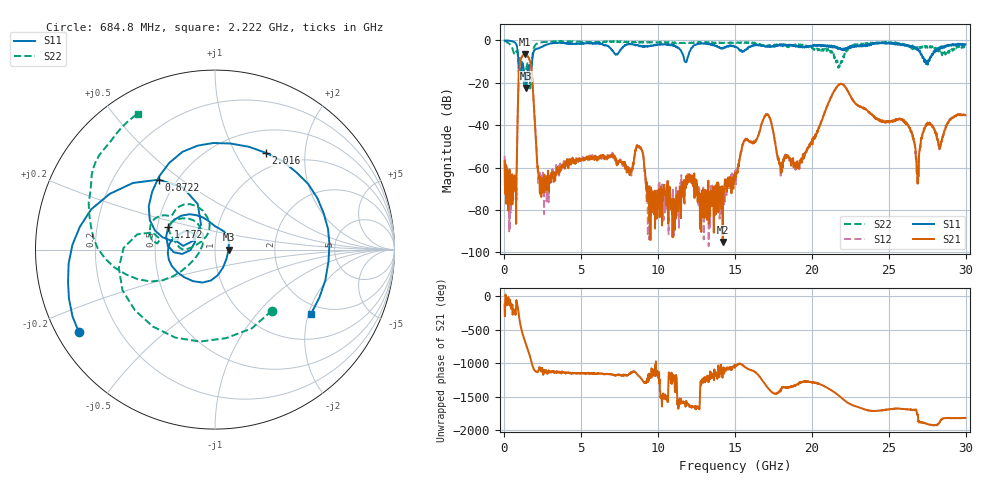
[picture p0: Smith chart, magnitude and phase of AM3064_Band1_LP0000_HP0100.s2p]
# Hz S DB R 50.0
!freq dBS11 angS11 dBS21 angS21 dBS12 angS12 dBS22 angS22
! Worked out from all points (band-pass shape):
!   1600 points, 10 MHz to 29.98 GHz, reference 50 ohm
!   highest |S21| = -6.49 dB at 1.322 GHz (marker M1); lowest = -95.1 dB at 14.2 GHz (marker M2)
!   |S21| within 3 dB of the highest: 1.042 GHz to 1.648 GHz (606 MHz wide, 45.1 % of centre)
!   lowest |S11| = -22.4 dB at 1.416 GHz (marker M3), VSWR 1.16, Z = 58.2 - j0.0524 ohm
!   |S11| at or under -10 dB: 901.9 MHz to 1.797 GHz (894.8 MHz wide, 66.3 % of centre); 11.74 GHz to 11.84 GHz (104.5 MHz wide, 0.887 % of centre); 27.39227 GHz to 27.45925 GHz (66.98 MHz wide, 0.244 % of centre)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
!   |S22| runs from -22.6 to -0.2 dB; largest |S21 - S12| = 0.0058
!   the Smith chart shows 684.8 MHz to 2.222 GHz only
!   S11 on the Smith chart (normalised r, x): 684.8 MHz: 0.06, -0.28; 872.2 MHz: 0.40, +0.41; 1.172 GHz: 0.57, +0.16; 2.016 GHz: 0.78, +1.34; 2.222 GHz: 1.70, -2.08
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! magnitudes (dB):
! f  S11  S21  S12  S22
! 10 MHz  0.0  -56.8  -54.4  -0.2
! 684.8 MHz  -1.0  -64.2  -65.9  -6.7
! 872.2 MHz  -6.0  -31.5  -31.5  -7.1
! 1.172 GHz  -10.8  -7.4  -7.3  -10.8
! 1.322 GHz  -17.9  -6.5  -6.4  -19.3
! 1.416 GHz  -22.4  -6.7  -6.7  -13.5
! 1.734 GHz  -13.1  -12.5  -12.4  -15.5
! 2.016 GHz  -4.3  -43.5  -43.7  -2.1
! 2.222 GHz  -3.8  -64.0  -64.6  -1.2
! 5.015 GHz  -1.4  -56.0  -56.0  -0.6
! 8.745 GHz  -2.6  -50.4  -50.0  -1.1
! 10 GHz  -2.0  -74.5  -70.6  -0.9
! 14.2 GHz  -3.8  -95.1  -74.0  -1.2
! 15 GHz  -3.0  -62.9  -67.3  -1.3
! 17.03 GHz  -3.0  -34.9  -35.0  -2.7
! 17.95 GHz  -2.3  -58.9  -59.4  -2.0
! 19.99 GHz  -2.9  -47.5  -48.6  -3.4
! 21.85 GHz  -3.6  -20.5  -20.4  -12.1
! 25 GHz  -1.0  -37.9  -38.7  -1.2
! 26.87 GHz  -4.4  -67.6  -66.7  -3.2
! 27.51 GHz  -10.7  -38.9  -39.9  -3.5
! 29.98 GHz  -1.8  -35.2  -35.4  -3.3
